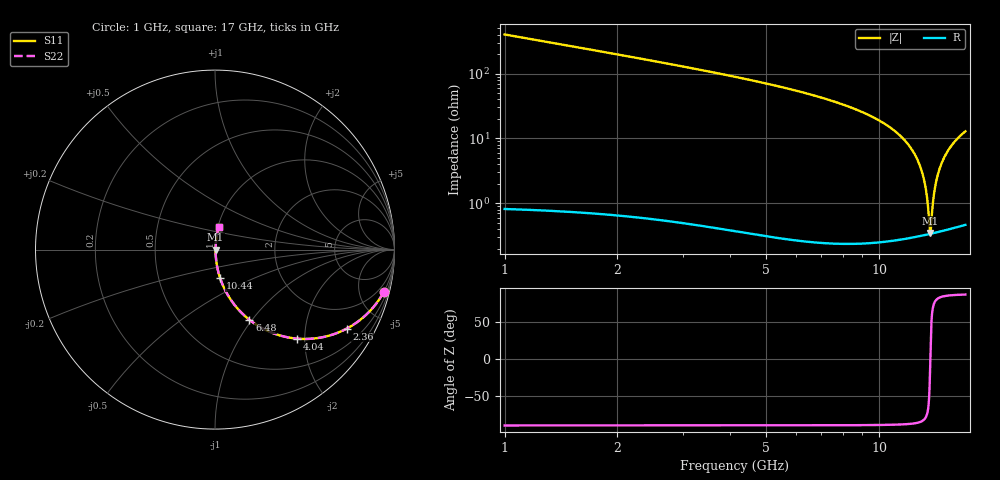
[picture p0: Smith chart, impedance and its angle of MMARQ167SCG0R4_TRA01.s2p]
! MMARQ167SCG0R4_TRA01  S-PARAMETER MODEL  ( General Type )
! Model Generated by TAIYO YUDEN Corporation (http://www.ty-top.com)
! Version 1.0
! TAIYO YUDEN Control No. 180601
! Copyright(c) 2018 TAIYO YUDEN CO.,LTD. All Rights Reserved.
! Product Description (link to TY-COMPAS)
! https://ds.yuden.co.jp/TYCOMPAS/or/detail?pn=MMARQ167SCG0R4ATRA01&u=M
! Products Name : Multilayer Ceramic Capacitors
! Characteristics :
!  Capacitance : 0.4 pF , Rated Voltage : 250V , TCC : CG / C0G
!  Case Size : 1.6 x 0.8 / 0.063 x 0.031 [mm/inch] , Thickness : 0.7 / 0.028 [mm/inch]
!  (Conditions: Temperature = 25 degC , DC Bias Current/Voltage = 0A / 0V)
! External Node Assignments :
!  1  o---| |---o  2
! GND o---------o GND
! Frequency Range : 1000MHz  -  17000MHz  [ 401 STEP ]
# MHz S RI R 50
! Freq[MHz].  S11 Real  S11 Imag  S21 Real  S21 Imag  S12 Real  S12 Imag  S22 Real  S22 Imag
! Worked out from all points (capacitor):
!   401 points, 1 GHz to 17 GHz, reference 50 ohm
!   read as one part in series: C = 394 fF near 1.08 GHz
!   lowest |Z| = 347 mohm at 13.68 GHz (marker M1)
!   series resonance near 13.7 GHz, so ESL is about 340 pH
!   S11 on the Smith chart (normalised r, x): 1 GHz: 1.02, -8.02; 2.36 GHz: 1.01, -3.32; 4.04 GHz: 1.01, -1.83; 6.48 GHz: 1.01, -0.97; 10.44 GHz: 1.01, -0.33; 17 GHz: 1.01, +0.26
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1000  0.9411 -0.2344  0.0589 0.2344  0.0589 0.2344  0.9411 -0.2344
1640  0.8541 -0.3516  0.1459 0.3516  0.1459 0.3516  0.8541 -0.3516
2360  0.7333 -0.4405  0.2667 0.4405  0.2667 0.4405  0.7333 -0.4405
3680  0.5099 -0.4979  0.4901 0.4979  0.4901 0.4979  0.5099 -0.4979
4040  0.4557 -0.496  0.5443 0.496  0.5443 0.496  0.4557 -0.496
6360  0.2011 -0.3982  0.7989 0.3982  0.7989 0.3982  0.2011 -0.3982
6480  0.1919 -0.3912  0.8081 0.3912  0.8081 0.3912  0.1919 -0.3912
9000  0.0635 -0.2392  0.9365 0.2392  0.9365 0.2392  0.0635 -0.2392
10440  0.0282 -0.1578  0.9718 0.1578  0.9718 0.1578  0.0282 -0.1578
11680  0.0116 -0.0934  0.9884 0.0934  0.9884 0.0934  0.0116 -0.0934
12480  0.00602 -0.0548  0.994 0.0548  0.994 0.0548  0.00602 -0.0548
13040  0.004 -0.029  0.996 0.029  0.996 0.029  0.004 -0.029
13360  0.00347 -0.0148  0.9965 0.0148  0.9965 0.0148  0.00347 -0.0148
13480  0.00338 -0.00951  0.9966 0.00951  0.9966 0.00951  0.00338 -0.00951
13680  0.00336 -0.000853  0.9966 0.000853  0.9966 0.000853  0.00336 -0.000853
13760  0.00339 0.00257  0.9966 -0.00257  0.9966 -0.00257  0.00339 0.00257
13920  0.00352 0.00937  0.9965 -0.00937  0.9965 -0.00937  0.00352 0.00937
14040  0.00368 0.0144  0.9963 -0.0144  0.9963 -0.0144  0.00368 0.0144
14360  0.00435 0.0276  0.9957 -0.0276  0.9957 -0.0276  0.00435 0.0276
14800  0.0058 0.0453  0.9942 -0.0453  0.9942 -0.0453  0.0058 0.0453
15360  0.00847 0.067  0.9915 -0.067  0.9915 -0.067  0.00847 0.067
17000  0.0207 0.1254  0.9793 -0.1254  0.9793 -0.1254  0.0207 0.1254
